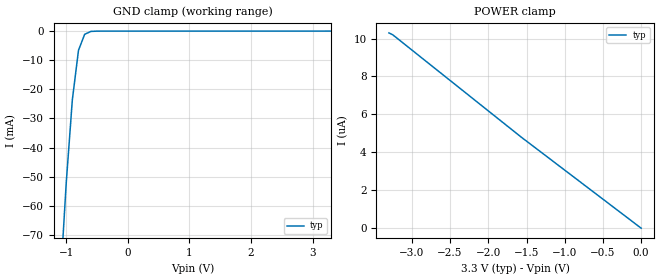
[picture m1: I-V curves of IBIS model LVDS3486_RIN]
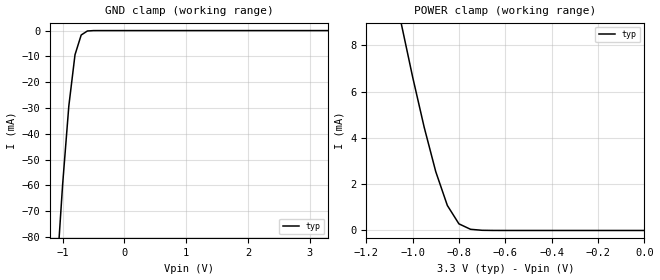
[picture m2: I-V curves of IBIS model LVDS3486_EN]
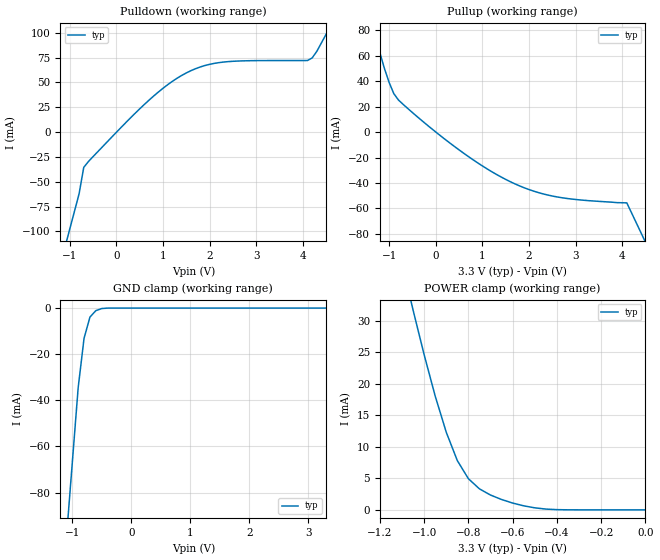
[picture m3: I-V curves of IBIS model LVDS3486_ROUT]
|   Texas Instruments Incorporated
|   Data Transmissions Products
|   IBIS Model for SN65LVDS3486
|   16D SOIC Package
[IBIS Ver]   2.1
[Comment char]   |_char
[File name]   lvds3486.ibs
[File Rev]   2.0
[Date]   10Feb98
[Source]   File originated at Texas Instruments Incorporated.
   Data Transmission Products Group. All data based on
   Bench Measurements.
[Notes]
[Disclaimer]
(C) Copyright Texas Instruments Incorporated 1997
   All rights reserved
  Texas Instruments Incorporated hereby grants the user of this IBIS
model a non-exclusive, nontransferable license to use this IBIS model
under the following terms.  Before using this IBIS model, the user
should read this license.  If the user does not accept these terms,
the IBIS model should be returned to Texas Instruments within 30 days.
  The user is granted this license only to use the IBIS model and
is not granted rights to sell, load, rent, lease or license the IBIS
model in whole or in part, or in modified form to anyone other than
user.  User may modify the IBIS model to suit its specific applications
but rights to derivative works and such modifications shall belong to
Texas Instruments.
  This IBIS model is provided on an "AS IS" basis and Texas Instruments
makes absolutely no warranty with respect to the information contained
herein.  TEXAS INSTRUMENTS DISCLAIMS AND CUSTOMER WAIVES ALL WARRANTIES,
EXPRESS OR IMPLIED, INCLUDING WARRANTIES OF MERCHANTABILITY OR FITNESS
FOR A PARTICULAR PURPOSE. The entire risk as to quality and performance
is with the Customer. ACCORDINGLY, IN NO EVENT SHALL THE COMPANY BE LIABLE
FOR ANY DAMAGES, WHETHER IN CONTRACT OR TORT,INCLUDING ANY LOST PROFITS
OR OTHER INCIDENTAL, CONSEQUENTIAL, EXEMPLARY, OR PUNITIVE DAMAGES ARISING
OUT OF THE USE OR APPLICATION OF THE IBIS model provided in this package.
Further, Texas Instruments reserves the right to discontinue or make changes
without notice to any product herein to improve reliability, function, or
design. Texas Instruments does not convey any license under patent rights
or any other intellectual property rights, including those of third parties.
Contact Texas Instruments at ATTN:DATA TRANSMISSIONS
Thomas Fisher 8505 Forest Lane, M/S 8710, Dallas, TX 75243
[Copyright]   Copyright 1997, Texas Instruments, All Rights Reserved
[Component]   SN65LVDS3486D
[Manufacturer]  Texas Instruments Incorporated
[Package]
|   typ   min   max
R_pkg   0.035   0.030   0.040
L_pkg   2.181nH   1.231nH   3.257nH
C_pkg   0.322pF   0.163pF   0.546pF
[Pin]   signal_name   model_name   R_pin   L_pin   C_pin
1   1B   LVDS3486_RIN   0.040   3.251n   0.546p
2   1A   LVDS3486_RIN   0.039   2.561n   0.393p
3   1Y   LVDS3486_ROUT   0.030   1.681n   0.186p
4   1,2EN   LVDS3486_EN   0.030   1.231n   0.163p
5   2Y   LVDS3486_ROUT   0.030   1.231n   0.163p
6   2A   LVDS3486_RIN   0.030   1.681n   0.186p
7   2B   LVDS3486_RIN   0.039   2.564n   0.393p
8   GND   GND   0.040   3.257n   0.545p
9   3B   LVDS3486_RIN   0.040   3.247n   0.546p
10   3A   LVDS3486_RIN   0.039   2.558n   0.394p
11   3Y   LVDS3486_ROUT   0.030   1.681n   0.187p
12   3,4EN   LVDS3486_EN   0.030   1.231n   0.163p
13   4Y   LVDS3486_ROUT   0.030   1.231n   0.163p
14   4A   LVDS3486_RIN   0.030   1.681n   0.187p
15   4B   LVDS3486_RIN   0.039   2.558n   0.394p
16   VCC   POWER   0.040   3.246n   0.546p
[Diff_pin]   inv_pin   vdiff   tdelay_typ   tdelay_min   tdelay_max
| The 'xA' pin is Diff_pin and the 'xB' pin is the inv_pin
2   1   100mV   0 0 0   | Vth  +/-100mV
6   7   100mV   0 0 0
10   9   100mV   0 0 0
14   15   100mV   0 0 0
| Models and submodels in the file (3): LVDS3486_RIN (Input), LVDS3486_EN (Input), LVDS3486_ROUT (3-state)
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|   Receiver Input  MODEL
[Model]   LVDS3486_RIN
Model_type   Input
|Signals   1A,1B,2A,2B,3A,3B,4A,4B
Vinh = 2.0
Vinl = 0.8
|   typ   min   max
C_comp   1.0pF   NA   NA
|   typ   min   max
[Temperature Range]   25.0   NA   NA
[Voltage range]   3.3V   3.0V   3.6V
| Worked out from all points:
|   GND clamp passes 1 mA (typ) near -0.69 V on its own axis
[GND_clamp]
|   Voltage   I(typ)   I(min)   I(max)
-3.3V     -873.9mA   NA         NA
-1.1V     -88.23mA   NA         NA
-1V       -52.52mA   NA         NA
-900mV    -23.67mA   NA         NA
-800mV    -6.59mA    NA         NA
-700mV    -1.12mA    NA         NA
-600mV    -120uA     NA         NA
-500mV    -15.1uA    NA         NA
3.3V      474pA      NA         NA
[Power_clamp]
| Note that the[POWER_clamp]voltage table is referenced to Vcc
| and is calculated using Vtable=Vcc - Vmeasured.
|   Voltage   I(typ)   I(min)   I(max)
-3.3V     10.3uA     NA         NA
-3.25V    10.2uA     NA         NA
-1.55V    4.74uA     NA         NA
-1.5V     4.59uA     NA         NA
-50mV     149nA      NA         NA
0V        -3.35nA    NA         NA
|   Receiver Enable  MODEL
[Model]   LVDS3486_EN
Model_type   Input
|Signals   1,2EN;3,4EN
Vinh = 2.0
Vinl = 0.8
|   typ   min   max
C_comp   1.0pF   NA   NA
|   typ   min   max
[Temperature Range]   25.0   NA   NA
[Voltage range]   3.3V   3.0V   3.6V
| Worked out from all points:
|   GND clamp passes 1 mA (typ) near -0.65 V on its own axis
|   POWER clamp passes 1 mA (typ) near -0.84 V on its own axis
[GND_clamp]
|   Voltage   I(typ)   I(min)   I(max)
-3.3V     -895.7mA   NA         NA
-1.1V     -95.97mA   NA         NA
-1V       -59.62mA   NA         NA
-900mV    -29.24mA   NA         NA
-800mV    -9.37mA    NA         NA
-700mV    -1.72mA    NA         NA
-600mV    -160uA     NA         NA
-500mV    -4.9uA     NA         NA
-400mV    -110nA     NA         NA
3.3V      3.96nA     NA         NA
[Power_clamp]
| Note that the[POWER_clamp]voltage table is referenced to Vcc
| and is calculated using Vtable=Vcc - Vmeasured.
|   Voltage   I(typ)   I(min)   I(max)
-3.3V     142mA      NA         NA
-1.05V    8.99mA     NA         NA
-1V       6.64mA     NA         NA
-950mV    4.46mA     NA         NA
-900mV    2.54mA     NA         NA
-850mV    1.08mA     NA         NA
-800mV    286uA      NA         NA
-750mV    51uA       NA         NA
-700mV    7.83uA     NA         NA
0V        1.77nA     NA         NA
|   Receiver Output  MODEL
[Model]   LVDS3486_ROUT
Model_type   3-state
| Signals   1Y,2Y,3Y,4Y
Vmeas = 1.5V   |Reference voltage for timing measurements
Cref = 8pF   |Timing specification test load capacitance value
Vref = 0   |Timing specification test load voltage; GND
| variable   typ   min   max
C_comp   1.0pF   NA   NA
|   typ   min   max
[Temperature Range]   25.0   NA   NA
[Voltage range]   3.3V   3.0V   3.6V
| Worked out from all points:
|   slope of the pulldown table from 0 to 0.495 V, typ, clamps not added: 21.2 ohm
|   slope of the pullup table from 0 to 0.495 V, typ, clamps not added: 35.5 ohm
|   GND clamp passes 1 mA (typ) near -0.59 V on its own axis
|   POWER clamp passes 1 mA (typ) near -0.59 V on its own axis
[Pulldown]
|   Voltage   I(typ)   I(min)   I(max)
-3.3V     -505.4mA   NA         NA
-900mV    -79.93mA   NA         NA
-800mV    -62.2mA    NA         NA
-700mV    -35.56mA   NA         NA
-600mV    -29.67mA   NA         NA
800mV     36.29mA    NA         NA
1.6V      61.86mA    NA         NA
2.4V      70.98mA    NA         NA
4.1V      72.09mA    NA         NA
4.2V      74.6mA     NA         NA
4.4V      89.79mA    NA         NA
6.6V      279.1mA    NA         NA
[Pullup]
|   Voltage   I(typ)   I(min)   I(max)
| Note that the[Pullup]voltage table is referenced to Vcc
| and is calculated using Vtable=Vcc - Vmeasured.
-3.3V     394.8mA    NA         NA
-1.4V     92.99mA    NA         NA
-1.3V     77.11mA    NA         NA
-1.2V     62.52mA    NA         NA
-1V       38.96mA    NA         NA
-800mV    25.22mA    NA         NA
600mV     -16.65mA   NA         NA
1.7V      -40.76mA   NA         NA
2.6V      -51.01mA   NA         NA
4.1V      -55.7mA    NA         NA
4.2V      -63.43mA   NA         NA
6.6V      -249mA     NA         NA
| Output in High Impedance (off)
[GND_clamp]
|   Voltage   I(typ)   I(min)   I(max)
-3.3V     -818.5mA   NA         NA
-1.1V     -99.97mA   NA         NA
-1V       -67.31mA   NA         NA
-900mV    -34.61mA   NA         NA
-800mV    -13.09mA   NA         NA
-700mV    -3.91mA    NA         NA
-600mV    -1.1mA     NA         NA
-500mV    -200uA     NA         NA
-400mV    -12.1uA    NA         NA
3.3V      797pA      NA         NA
[POWER_clamp]
|   Voltage   I(typ)   I(min)   I(max)
| Note that the [POWER_clamp] voltage table is referenced to Vcc
| and is calculated using Vtable = Vcc - Vmeasured.
| Outputs in Tri-state.
-3.3V     412.8mA    NA         NA
-1.1V     39.15mA    NA         NA
-1.05V    31.72mA    NA         NA
-1V       24.63mA    NA         NA
-950mV    18.07mA    NA         NA
-900mV    12.32mA    NA         NA
-850mV    7.816mA    NA         NA
-800mV    4.946mA    NA         NA
-750mV    3.33mA     NA         NA
-650mV    1.642mA    NA         NA
-500mV    320uA      NA         NA
0V        803pA      NA         NA
[Ramp]
|   typ   min   max
dV/dt_r   2.0v/512ps   NA   NA
dV/dt_f   2.0v/385ps   NA   NA
R_load = 1MOhm   | Represents an open
